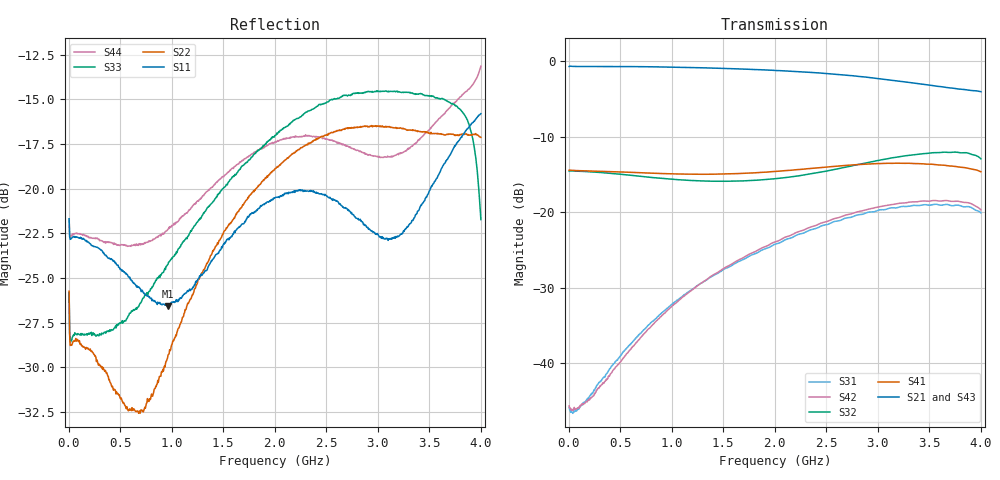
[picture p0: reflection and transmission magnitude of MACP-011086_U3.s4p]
!Agilent Technologies,E5071C,MY46110647,A.11.31
!Date: Thu Jul 09 12:06:40 2020 DD
!Data & Calibration Information:
!MACP-011086 soldered onto PT-0010289 with SMA connectors, calibration PCB PT-0003654. Port1 (pin1) Port2 (pin5) Port3 (pin4) Port4 (pin3)
!Freq	S11:SOLT4(ON)	S12:SOLT4(ON)	S13:SOLT4(ON)	S14:SOLT4(ON)
!	S21:SOLT4(ON)	S22:SOLT4(ON)	S23:SOLT4(ON)	S24:SOLT4(ON)
!	S31:SOLT4(ON)	S32:SOLT4(ON)	S33:SOLT4(ON)	S34:SOLT4(ON)
!	S41:SOLT4(ON)	S42:SOLT4(ON)	S43:SOLT4(ON)	S44:SOLT4(ON)
!PortZ  Port1:50+j0  Port2:50+j0  Port3:50+j0  Port4:50+j0
!Above PortZ is port z conversion or system Z0 setting when saving the data.
!When reading, reference impedance value at option line is always used.
# Hz S MA R 50
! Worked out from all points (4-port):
!   800 points, 5 MHz to 4 GHz, reference 50 ohm
!   strongest paths, dB at 5 MHz, 1.005 GHz, 2.005 GHz, 3.005 GHz, 4 GHz:
!     S21: -0.7, -0.8, -1.2, -2.3, -4.0
!     S43: -0.7, -0.9, -1.4, -2.5, -5.1
!     S41: -14.5, -14.9, -14.6, -13.6, -14.6
!     S32: -14.6, -15.6, -15.6, -13.1, -12.9
!     S42: -45.7, -32.4, -23.9, -19.3, -19.7
!     S31: -45.9, -32.2, -24.2, -19.7, -20.1
!   lowest |S11| = -26.6 dB at 960 MHz (marker M1), VSWR 1.10, Z = 51 + j4.63 ohm
!   |S11| at or under -10 dB: start of sweep to end of sweep
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5000000  0.08238 157.6  0.9235 1.8  0.004736 176.3  0.1895 -178.6
         0.9231 1.8  0.0517 140.6  0.1873 2.1  0.004708 175.8
         0.005099 171.6  0.187 2.0  0.05128 142.3  0.9221 1.7
         0.1894 -178.8  0.005206 174.3  0.922 1.7  0.08226 158.5
5.9e8  0.05642 125.6  0.9213 -14.4  0.01284 170.1  0.1836 144.3
       0.9211 -14.4  0.02421 99.6  0.176 -10.4  0.01187 151.7
       0.01314 169.0  0.1759 -10.3  0.04485 90.9  0.9169 -14.9
       0.1837 144.2  0.01215 152.2  0.917 -14.9  0.06916 113.6
9.6e8  0.04691 75.1  0.9149 -23.7  0.02258 142.4  0.1798 123.6
       0.9151 -23.7  0.03362 28.9  0.1661 -13.5  0.02219 128.2
       0.02319 141.7  0.1661 -13.5  0.06138 50.6  0.9083 -24.4
       0.1798 123.6  0.02238 128.3  0.9082 -24.4  0.0767 69.7
1.76e9  0.08487 -4.4  0.8834 -44.0  0.05053 88.6  0.1821 82.9
        0.8833 -44.0  0.09586 -20.8  0.1618 -15.0  0.05261 81.6
        0.05151 89.4  0.1619 -14.9  0.1208 3.3  0.8724 -45.0
        0.1817 83.0  0.05296 81.5  0.8718 -45.0  0.1235 12.6
2.78e9  0.08346 -27.4  0.7975 -70.6  0.09642 23.0  0.2071 26.3
        0.7979 -70.7  0.1484 -49.2  0.205 -21.1  0.09964 21.9
        0.09481 24.8  0.205 -21.4  0.1846 -32.3  0.7853 -72.2
        0.206 26.6  0.09944 21.5  0.7813 -72.2  0.1287 -6.3
3.785e9  0.1361 17.5  0.6568 -93.6  0.1167 -58.6  0.2014 -45.1
         0.6542 -93.7  0.1408 -63.8  0.2501 -53.3  0.1201 -55.1
         0.1111 -57.1  0.2484 -53.8  0.1677 -56.2  0.6318 -97.8
         0.1992 -44.5  0.1179 -55.4  0.6264 -97.3  0.1783 22.7
4e9  0.1621 14.9  0.6331 -97.8  0.1049 -80.0  0.1878 -60.9
     0.6282 -98.0  0.1392 -67.1  0.2277 -64.1  0.106 -75.0
     0.09901 -78.7  0.2255 -64.8  0.08192 -60.3  0.5574 -104.6
     0.1852 -60.4  0.1037 -75.9  0.553 -104.1  0.2201 29.4
